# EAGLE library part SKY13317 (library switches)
Description: Device for SKY13317-373LF, an RF switch from Skyworks Inc.
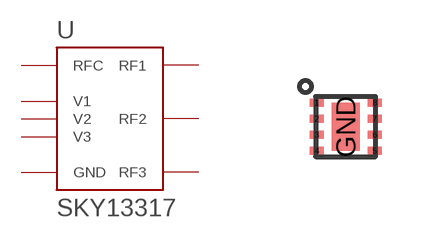
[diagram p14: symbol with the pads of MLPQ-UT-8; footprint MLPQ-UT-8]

Designator prefix U

## SKY13317 (DATASHEET: http://www.skyworksinc.com/uploads/documents/SKY13317_373LF_200914K.pdf; DESCRIPTION: IC SWITCH RF SP3T 8-MLP; DIGIKEY: 863-1056-1-ND; MANUFACTURER: Skyworks Solutions Inc.; MPN: SKY13317-373LF)  [MLPQ-UT-8]
1  RFC
3  V1
4  RF1
5  RF2
6  V2
7  V3
8  RF3
GND  GND  pwr

## Footprint MLPQ-UT-8 (pad centres in mm)
MLP 8-pin 1.5 x 1.5mm
smd 0.35 x 0.2: 1 -0.725,0.6; 2 -0.725,0.2; 3 -0.725,-0.2; 4 -0.725,-0.6; 5 0.725,-0.6; 6 0.725,-0.2; 7 0.725,0.2; 8 0.725,0.6
smd 0.7 x 1.2: GND 0,0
